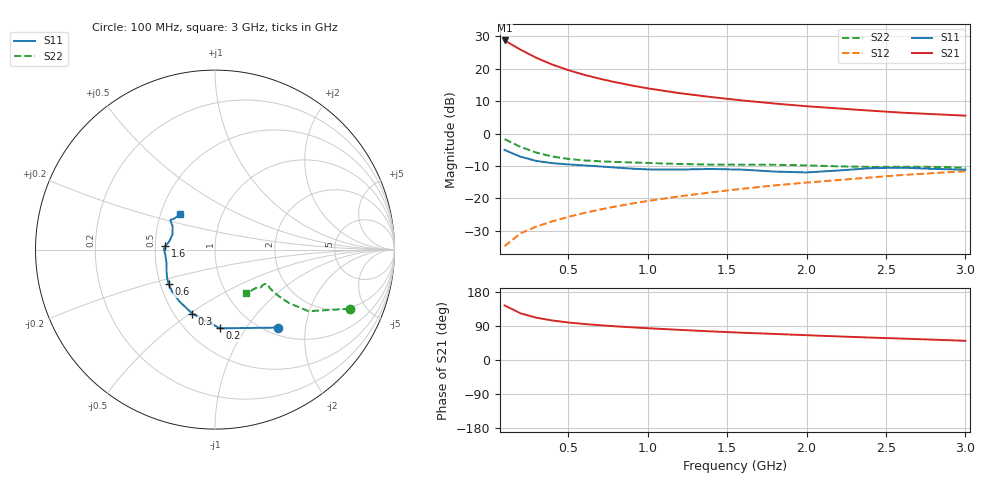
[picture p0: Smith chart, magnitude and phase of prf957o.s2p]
! Filename:  PRF957O.S2P  Version:  3.0
! Philips part #:  PRF957  Date:  Nov 1998
! Bias condition:  Vce=6V, Ic=15mA
#  MHz  S  MA  R 50
! Freq  S11  S21  S12  S22
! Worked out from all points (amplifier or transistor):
!   20 points, 100 MHz to 3 GHz, reference 50 ohm
!   highest |S21| = 28.7 dB at 100 MHz (marker M1)
!   |S21| within 3 dB of that: start of sweep to 206.3 MHz
!   unconditionally stable (mu >= 1): 911.7 MHz to end of sweep
!   at 400 MHz: K = 0.81, MSG = 24.2 dB, |S12| = -27.1 dB
!   at 1.2 GHz: K = 1.03, MAG = 14.8 dB, |S12| = -19.4 dB
!   at 3 GHz: K = 1.03, MAG = 7.5 dB, |S12| = -11.6 dB
!   lowest NFmin = 1.44 dB at 500 MHz
!   S11 on the Smith chart (normalised r, x): 100 MHz: 1.13, -1.42; 200 MHz: 0.71, -0.77; 300 MHz: 0.61, -0.51; 600 MHz: 0.55, -0.24; 1.6 GHz: 0.57, +0.02; 3 GHz: 0.63, +0.27
100  0.5582 -51.1  27.37 144.0  0.0183 70.1  0.8205 -23.7
200  0.4396 -86.4  19.74 123.2  0.02888 64.2  0.6239 -33.4
300  0.3783 -109.6  14.75 111.6  0.03678 64.0  0.5083 -35.9
400  0.3497 -125.1  11.62 104.3  0.04422 65.7  0.4435 -36.1
500  0.3343 -135.6  9.549 99.1  0.05181 67.6  0.4068 -35.9
600  0.3227 -143.2  8.095 95.1  0.05947 69.2  0.3855 -35.5
700  0.3112 -149.0  7.015 91.8  0.06724 70.5  0.3733 -35.0
800  0.2989 -154.3  6.189 88.9  0.07509 71.6  0.3654 -34.5
900  0.2877 -159.6  5.525 86.2  0.08307 72.5  0.3587 -34.0
1000  0.28 -165.0  4.996 83.9  0.09114 73.1  0.3524 -33.7
1200  0.2785 -174.5  4.209 79.6  0.1075 73.8  0.3399 -34.1
1400  0.2846 179.6  3.666 75.5  0.124 74.1  0.3319 -36.2
1600  0.2776 175.9  3.24 71.9  0.141 74.2  0.3311 -38.4
1800  0.2591 170.0  2.907 68.8  0.1585 74.0  0.3305 -39.6
2000  0.2515 160.1  2.646 65.5  0.1753 73.8  0.3236 -40.8
2200  0.2692 151.2  2.444 62.2  0.192 73.4  0.3121 -43.3
2400  0.292 147.5  2.262 59.3  0.2098 72.7  0.3058 -47.1
2600  0.298 146.1  2.104 56.5  0.2293 71.9  0.3072 -50.6
2800  0.2853 142.8  1.995 53.6  0.2454 71.5  0.3067 -52.6
3000  0.2774 135.1  1.892 50.7  0.263 71.0  0.2986 -54.6
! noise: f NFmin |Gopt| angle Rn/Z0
500  1.44  0.08  43  0.15
800  1.57  0.14  98  0.2
900  1.72  0.17  102  0.14
1000  1.71  0.17  96  0.225
1500  1.69  0.31  133  0.13
2000  2.05  0.29  -155  0.16
